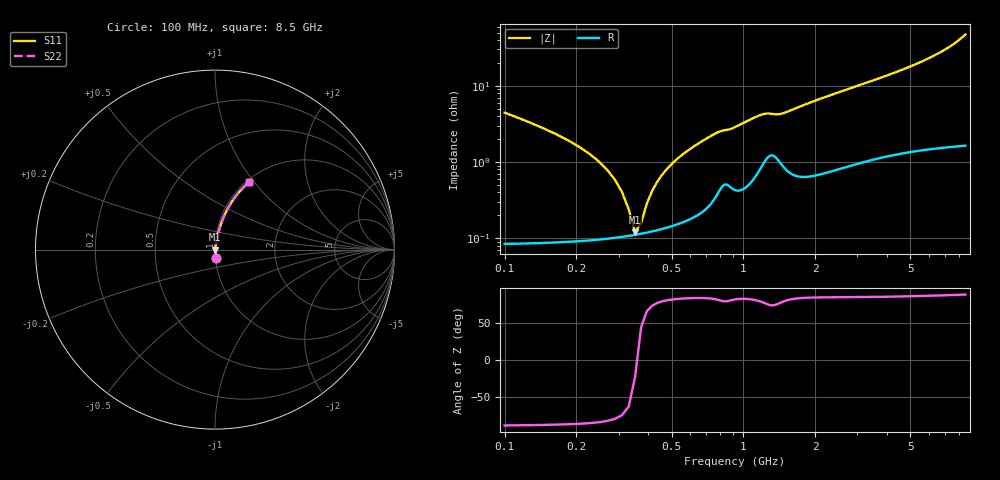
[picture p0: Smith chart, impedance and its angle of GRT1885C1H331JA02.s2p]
!Murata Part Number: GRT1885C1H331JA02
!These Parameters are Measured in Series Mode Connection
!Data Generated on Jun 19, 2026
!  o--ll--o
!Port1  Port2
!  o------o
!Operation Temp=25[degC], DC Bias Voltage=0[V]
!Freq. Start=100[MHz] Stop=9[GHz] 401[Steps]
# Hz S RI R 50
!Freq.(Hz) S11(Real) S11(Imag) S21(Real) S21(Imag) S12(Real) S12(Imag) S22(Real) S22(Imag)
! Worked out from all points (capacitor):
!   401 points, 100 MHz to 8.5 GHz, reference 50 ohm
!   read as one part in series: C = 330 pF near 142 MHz
!   lowest |Z| = 120 mohm at 352 MHz (marker M1)
!   series resonance near 358.2 MHz, so ESL is about 600 pH
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1e8  0.00281 -0.0443  0.9972 0.0443  0.9972 0.0443  0.00281 -0.0443
1.42e8  0.00168 -0.0286  0.9983 0.0286  0.9983 0.0286  0.00168 -0.0286
2.47e8  0.00106 -0.0102  0.9989 0.0102  0.9989 0.0102  0.00106 -0.0102
2.89e8  0.00105 -0.00583  0.999 0.00583  0.999 0.00583  0.00105 -0.00583
3.1e8  0.00106 -0.00391  0.9989 0.00391  0.9989 0.00391  0.00106 -0.00391
3.31e8  0.00108 -0.00213  0.9989 0.00213  0.9989 0.00213  0.00108 -0.00213
3.52e8  0.00111 -0.000464  0.9989 0.000464  0.9989 0.000464  0.00111 -0.000464
3.73e8  0.00115 0.0011  0.9989 -0.0011  0.9989 -0.0011  0.00115 0.0011
3.94e8  0.00119 0.00259  0.9988 -0.00259  0.9988 -0.00259  0.00119 0.00259
4.36e8  0.0013 0.00537  0.9987 -0.00537  0.9987 -0.00537  0.0013 0.00537
4.99e8  0.00152 0.00919  0.9985 -0.00919  0.9985 -0.00919  0.00152 0.00919
5.83e8  0.00191 0.0139  0.9981 -0.0139  0.9981 -0.0139  0.00191 0.0139
7.09e8  0.00296 0.0206  0.997 -0.0206  0.997 -0.0206  0.00296 0.0206
7.93e8  0.00479 0.0245  0.9952 -0.0245  0.9952 -0.0245  0.00479 0.0245
1.171e9  0.00946 0.0396  0.9905 -0.0396  0.9905 -0.0396  0.00946 0.0396
1.507e9  0.00979 0.0435  0.9902 -0.0435  0.9902 -0.0435  0.00979 0.0435
2.095e9  0.0112 0.0659  0.9888 -0.0659  0.9888 -0.0659  0.0112 0.0659
2.914e9  0.0181 0.0937  0.9819 -0.0937  0.9819 -0.0937  0.0181 0.0937
4.3e9  0.0331 0.1419  0.9669 -0.1419  0.9669 -0.1419  0.0331 0.1419
5.707e9  0.0564 0.1996  0.9436 -0.1996  0.9436 -0.1996  0.0564 0.1996
7.114e9  0.099 0.2745  0.901 -0.2745  0.901 -0.2745  0.099 0.2745
8.5e9  0.1905 0.3757  0.8095 -0.3757  0.8095 -0.3757  0.1905 0.3757
